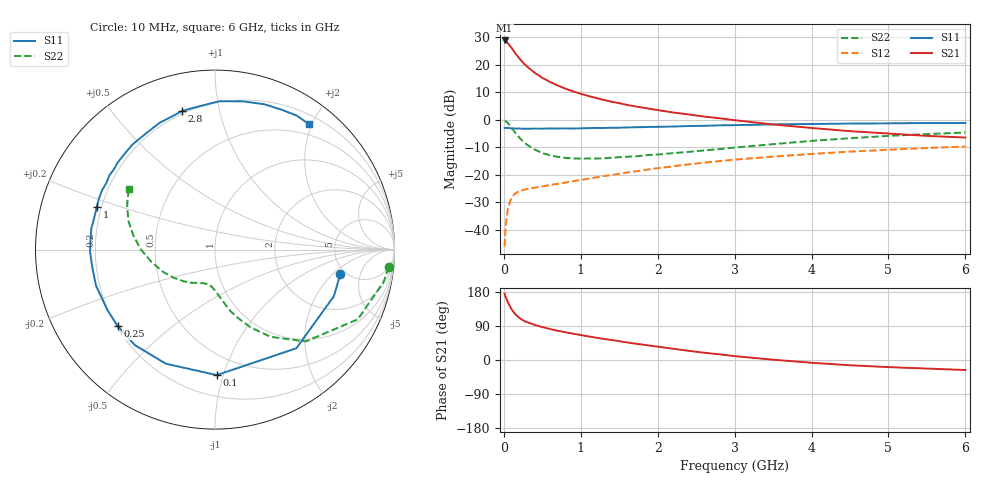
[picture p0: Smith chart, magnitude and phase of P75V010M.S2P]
! SIEMENS Small Signal Semiconductors
! BFP196
! Si NPN RF Bipolar Junction Transistor in SOT143
! VCE = 5 V  IC = 10 mA
! Common Emitter S-Parameters:  May  1996
# GHz  S  MA  R  50
!  f  S11  S21  S12  S22
! GHz  MAG  ANG  MAG  ANG  MAG  ANG  MAG  ANG
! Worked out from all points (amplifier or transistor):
!   36 points, 10 MHz to 6 GHz, reference 50 ohm
!   highest |S21| = 28.9 dB at 10 MHz (marker M1)
!   |S21| within 3 dB of that: start of sweep to 107.8 MHz
!   unconditionally stable (mu >= 1): 884.9 MHz to 3.285 GHz
!   at 250 MHz: K = 0.39, MSG = 23.2 dB, |S12| = -25.6 dB
!   at 1.4 GHz: K = 1.14, MAG = 11.1 dB, |S12| = -20.1 dB
!   at 6 GHz: K = 0.96, MSG = 1.6 dB, |S12| = -9.7 dB
!   S11 on the Smith chart (normalised r, x): 10 MHz: 4.51, -2.48; 100 MHz: 0.35, -0.95; 250 MHz: 0.21, -0.33; 1 GHz: 0.18, +0.17; 2.8 GHz: 0.19, +0.77; 6 GHz: 0.33, +1.96
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0.01  0.7115 -11.0  27.92 175.1  0.005 84.0  0.9734 -5.8
0.02  0.7114 -21.4  27.08 168.5  0.0099 79.9  0.9561 -10.9
0.05  0.7125 -50.5  25.17 153.5  0.0235 66.2  0.8855 -26.0
0.1  0.6992 -89.2  20.51 133.8  0.0382 51.3  0.7196 -45.3
0.15  0.6923 -113.3  16.19 120.4  0.0461 42.6  0.5771 -57.4
0.2  0.6947 -130.0  13.25 111.4  0.0502 37.5  0.4769 -65.4
0.25  0.6891 -142.0  10.98 104.7  0.0527 34.7  0.4024 -71.4
0.3  0.6877 -150.6  9.376 100.0  0.0551 33.6  0.3545 -75.8
0.4  0.6926 -163.1  7.232 92.8  0.0581 32.9  0.2877 -81.7
0.5  0.6906 -171.7  5.824 86.9  0.0614 33.4  0.2481 -86.5
0.6  0.696 -178.9  4.903 81.8  0.065 35.0  0.2256 -90.5
0.7  0.6958 175.1  4.23 77.1  0.0682 36.7  0.212 -93.8
0.8  0.6989 170.2  3.7 73.3  0.0721 38.0  0.2028 -97.0
1  0.7001 160.2  2.983 65.9  0.0804 40.4  0.1964 -102.2
1.1  0.7064 156.2  2.719 62.3  0.0847 41.3  0.1972 -105.2
1.6  0.7275 138.3  1.872 46.4  0.1099 43.7  0.2125 -118.9
2.2  0.7548 119.7  1.361 29.7  0.1426 42.2  0.2476 -134.0
2.8  0.7933 103.4  1.07 15.0  0.1771 37.7  0.2933 -151.3
3.5  0.8268 88.4  0.825 0.8  0.2139 30.6  0.3606 -168.9
4.5  0.855 71.3  0.622 -13.9  0.2637 19.9  0.4627 170.0
5.5  0.8744 58.7  0.51 -22.6  0.3071 8.6  0.5507 152.7
6  0.8739 53.0  0.476 -26.4  0.3264 2.4  0.5881 144.8
